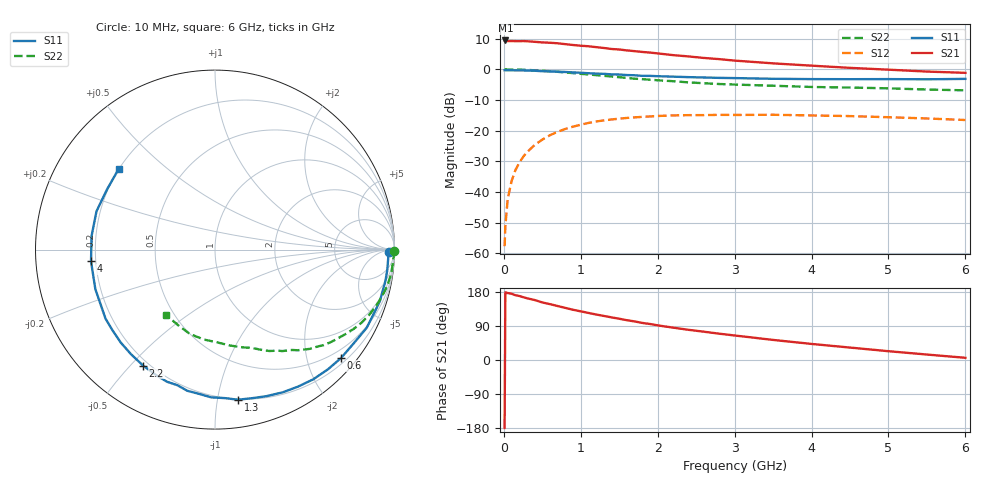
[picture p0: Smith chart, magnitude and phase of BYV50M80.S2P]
! SIEMENS Small Signal Semiconductors
! BFY420
! Si NPN RF SIEGET Grounded Emitter Transistor in MICRO-X
! VCE = 0.5 V  IC = 0.8 mA
! Common Emitter S-Parameters:  October  1996
# GHz  S  MA  R  50
!  f  S11  S21  S12  S22
! GHz  MAG  ANG  MAG  ANG  MAG  ANG  MAG  ANG
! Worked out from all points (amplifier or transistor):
!   36 points, 10 MHz to 6 GHz, reference 50 ohm
!   highest |S21| = 9.4 dB at 20 MHz (marker M1)
!   |S21| within 3 dB of that: start of sweep to 1.517 GHz
!   unconditionally stable (mu >= 1): 4.644 GHz to end of sweep
!   at 250 MHz: K = 0.04, MSG = 18.9 dB, |S12| = -28.6 dB
!   at 1.4 GHz: K = 0.26, MSG = 11.5 dB, |S12| = -16.4 dB
!   at 6 GHz: K = 1.34, MAG = 4.2 dB, |S12| = -16.5 dB
!   S11 on the Smith chart (normalised r, x): 10 MHz: 53, -19; 600 MHz: 0.31, -2.66; 1.3 GHz: 0.19, -1.15; 2.2 GHz: 0.18, -0.54; 4 GHz: 0.18, -0.05; 6 GHz: 0.20, +0.35
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0.01  0.9672 -0.7  2.955 -179.3  0.0013 93.6  0.9977 -0.4
0.02  0.967 -1.5  2.966 178.7  0.0028 89.3  0.9999 -0.8
0.05  0.966 -3.5  2.895 176.7  0.0076 89.7  0.9963 -2.0
0.1  0.9666 -6.9  2.9 174.9  0.0149 84.7  0.9939 -4.0
0.15  0.9654 -10.4  2.891 170.9  0.0226 82.3  0.992 -6.0
0.2  0.9622 -13.6  2.883 169.0  0.0298 80.8  0.9912 -7.9
0.3  0.9564 -20.4  2.88 163.0  0.0444 76.5  0.9811 -11.9
0.4  0.9508 -27.3  2.821 158.3  0.0582 71.7  0.966 -15.8
0.5  0.9327 -34.1  2.754 151.9  0.0714 67.6  0.9497 -19.5
0.6  0.9263 -40.7  2.721 147.4  0.0843 63.4  0.9325 -23.0
0.8  0.9066 -52.9  2.579 137.4  0.1067 55.1  0.8899 -29.8
1.1  0.8653 -70.7  2.386 124.2  0.1336 44.2  0.8261 -38.6
1.3  0.8462 -81.3  2.236 116.3  0.147 37.7  0.7844 -43.6
1.5  0.8237 -91.4  2.112 108.9  0.1569 31.7  0.7451 -48.4
1.8  0.7841 -105.5  1.926 97.8  0.168 24.2  0.6927 -54.2
2.2  0.7605 -121.8  1.708 85.4  0.1772 15.2  0.6411 -61.8
2.8  0.7266 -142.0  1.47 69.4  0.181 5.0  0.5768 -71.3
3.5  0.7021 -161.7  1.254 53.0  0.1816 -4.1  0.5405 -81.2
4  0.6939 -174.6  1.15 42.4  0.177 -9.8  0.5162 -89.0
4.5  0.6918 173.7  1.059 32.8  0.1727 -14.9  0.505 -96.9
5.5  0.6887 150.8  0.921 14.4  0.158 -22.0  0.4685 -116.0
6  0.6998 140.1  0.878 5.8  0.1491 -23.6  0.4552 -126.7
